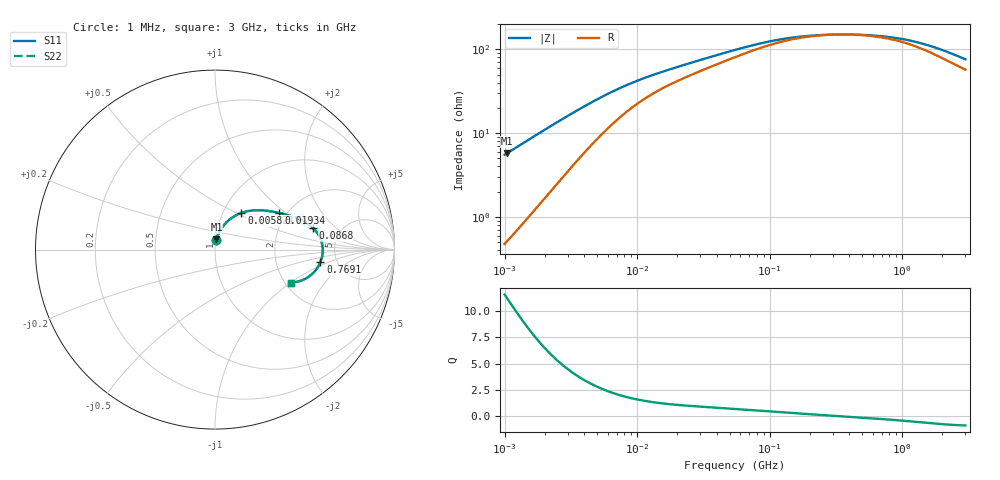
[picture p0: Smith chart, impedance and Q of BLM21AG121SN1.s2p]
! BLM21AG121SN1
# Hz S RI R 50
!Freq.(Hz) S11(Real) S11(Imag) S21(Real) S21(Imag) S12(Real) S12(Imag) S22(Real) S22(Imag)
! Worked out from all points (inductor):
!   401 points, 1 MHz to 3 GHz, reference 50 ohm
!   read as one part in series: L = 872 nH near 1.041 MHz
!   highest Q = 11.2 at 1.041 MHz (marker M1), where L = 876 nH
!   self-resonance near 348.2 MHz
!   S11 on the Smith chart (normalised r, x): 1 MHz: 1.01, +0.11; 5.821 MHz: 1.22, +0.53; 19.34 MHz: 1.81, +0.89; 86.8 MHz: 3.10, +1.10; 769.1 MHz: 3.70, -0.81; 3 GHz: 2.15, -1.00
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1000000  0.00772 0.0544  0.9923 -0.0544  0.9923 -0.0544  0.00772 0.0544
1040844  0.00829 0.0565  0.9917 -0.0565  0.9917 -0.0565  0.00829 0.0565
2182827  0.032 0.1113  0.968 -0.1113  0.968 -0.1113  0.032 0.1113
2888807  0.0522 0.1392  0.9478 -0.1392  0.9478 -0.1392  0.0522 0.1392
3823119  0.0822 0.1682  0.9178 -0.1682  0.9178 -0.1682  0.0822 0.1682
5820586  0.1468 0.2043  0.8532 -0.2043  0.8532 -0.2043  0.1468 0.2043
7110411  0.1833 0.2145  0.8167 -0.2145  0.8167 -0.2145  0.1833 0.2145
8861669  0.2246 0.2194  0.7754 -0.2194  0.7754 -0.2194  0.2246 0.2194
1.461624e7  0.3112 0.2131  0.6888 -0.2131  0.6888 -0.2131  0.3112 0.2131
1.934349e7  0.3539 0.205  0.6461 -0.205  0.6461 -0.205  0.3539 0.205
3.320783e7  0.4304 0.185  0.5696 -0.185  0.5696 -0.185  0.4304 0.185
5.477226e7  0.4953 0.1574  0.5047 -0.1574  0.5047 -0.1574  0.4953 0.1574
8.679508e7  0.5444 0.122  0.4556 -0.122  0.4556 -0.122  0.5444 0.122
1.375402e8  0.5776 0.0805  0.4224 -0.0805  0.4224 -0.0805  0.5776 0.0805
2.094008e8  0.5938 0.0429  0.4062 -0.0429  0.4062 -0.0429  0.5938 0.0429
4.135554e8  0.6001 -0.0144  0.3999 0.0144  0.3999 0.0144  0.6001 -0.0144
7.691493e8  0.5869 -0.0709  0.4131 0.0709  0.4131 0.0709  0.5869 -0.0709
8.005644e8  0.5851 -0.0749  0.4149 0.0749  0.4149 0.0749  0.5851 -0.0749
1.125055e9  0.5643 -0.1105  0.4357 0.1105  0.4357 0.1105  0.5643 -0.1105
1.519029e9  0.534 -0.142  0.466 0.142  0.466 0.142  0.534 -0.142
2.177892e9  0.4809 -0.1724  0.5191 0.1724  0.5191 0.1724  0.4809 -0.1724
3e9  0.4225 -0.1836  0.5775 0.1836  0.5775 0.1836  0.4225 -0.1836
